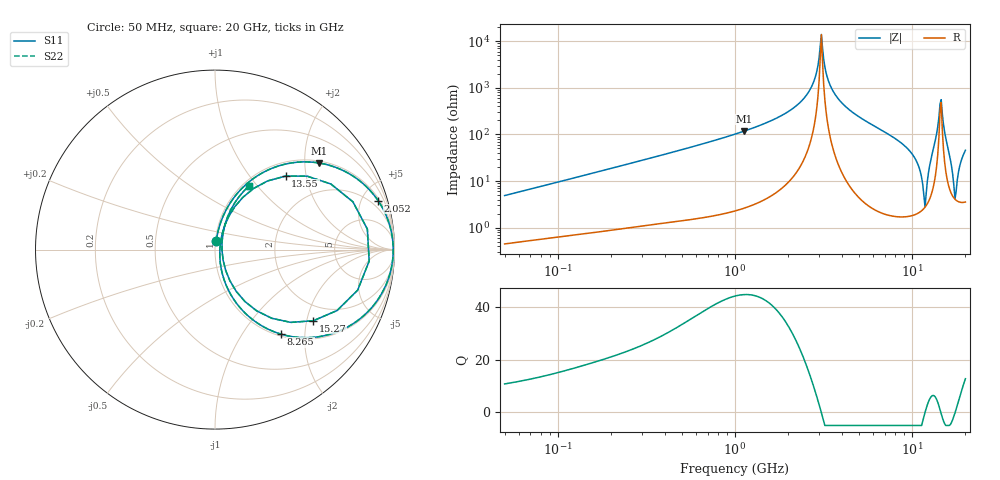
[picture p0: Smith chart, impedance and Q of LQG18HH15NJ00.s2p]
!Murata Part Number: LQG18HH15NJ00
!These Parameters are Measured in Series Mode Connection
!  o--[Z]--o
!Port1  Port2
!  o-------o
!Freq. Start=50[MHz] Stop=20[GHz], 401[Steps]
# Hz S RI R 50
!Freq.(Hz) S11(Real) S11(Imag) S21(Real) S21(Imag) S12(Real) S12(Imag) S22(Real) S22(Imag)
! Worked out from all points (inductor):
!   401 points, 50 MHz to 20 GHz, reference 50 ohm
!   read as one part in series: L = 15.3 nH near 51.52 MHz
!   highest Q = 44.9 at 1.127 GHz (marker M1), where L = 16.7 nH
!   self-resonance near 3.03 GHz
!   S11 on the Smith chart (normalised r, x): 50 MHz: 1.01, +0.10; 2.052 GHz: 1.21, +6.60; 8.265 GHz: 1.03, -1.51; 13.55 GHz: 1.26, +1.53; 15.27 GHz: 1.50, -2.19; 20 GHz: 1.07, +0.91
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5e7  0.00681 0.0482  0.9932 -0.0482  0.9932 -0.0482  0.00681 0.0482
1.364002e8  0.0232 0.1248  0.9768 -0.1248  0.9768 -0.1248  0.0232 0.1248
3.721004e8  0.1163 0.3036  0.8837 -0.3036  0.8837 -0.3036  0.1163 0.3036
1e9  0.5075 0.4888  0.4925 -0.4888  0.4925 -0.4888  0.5075 0.4888
1.127304e9  0.5804 0.4825  0.4196 -0.4825  0.4196 -0.4825  0.5804 0.4825
2.05233e9  0.9089 0.2724  0.0911 -0.2724  0.0911 -0.2724  0.9089 0.2724
2.728004e9  0.9849 0.0863  0.0151 -0.0863  0.0151 -0.0863  0.9849 0.0863
3.075291e9  0.9929 -0.000963  0.00706 0.000963  0.00706 0.000963  0.9929 -0.000963
3.415248e9  0.9869 -0.0793  0.0131 0.0793  0.0131 0.0793  0.9869 -0.0793
3.908127e9  0.9596 -0.1798  0.0404 0.1798  0.0404 0.1798  0.9596 -0.1798
7.442007e9  0.4908 -0.4907  0.5092 0.4907  0.5092 0.4907  0.4908 -0.4907
8.264682e9  0.3665 -0.4706  0.6335 0.4706  0.6335 0.4706  0.3665 -0.4706
1.050288e10  0.0895 -0.2533  0.9105 0.2533  0.9105 0.2533  0.0895 -0.2533
1.183995e10  0.0269 0.00142  0.9731 -0.00142  0.9731 -0.00142  0.0269 0.00142
1.276073e10  0.1103 0.239  0.8897 -0.239  0.8897 -0.239  0.1103 0.239
1.354865e10  0.3937 0.4097  0.6063 -0.4097  0.6063 -0.4097  0.3937 0.4097
1.438523e10  0.8489 0.1143  0.1511 -0.1143  0.1511 -0.1143  0.8489 0.1143
1.482269e10  0.7947 -0.2261  0.2053 0.2261  0.2053 0.2261  0.7947 -0.2261
1.527346e10  0.548 -0.3961  0.452 0.3961  0.452 0.3961  0.548 -0.3961
1.621653e10  0.1663 -0.2887  0.8337 0.2887  0.8337 0.2887  0.1663 -0.2887
1.747767e10  0.0392 -0.0069  0.9608 0.0069  0.9608 0.0069  0.0392 -0.0069
2e10  0.1911 0.3561  0.8089 -0.3561  0.8089 -0.3561  0.1911 0.3561
